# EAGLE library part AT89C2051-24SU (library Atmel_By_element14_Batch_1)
8-bit Microcontroller with 2K Bytes Flash
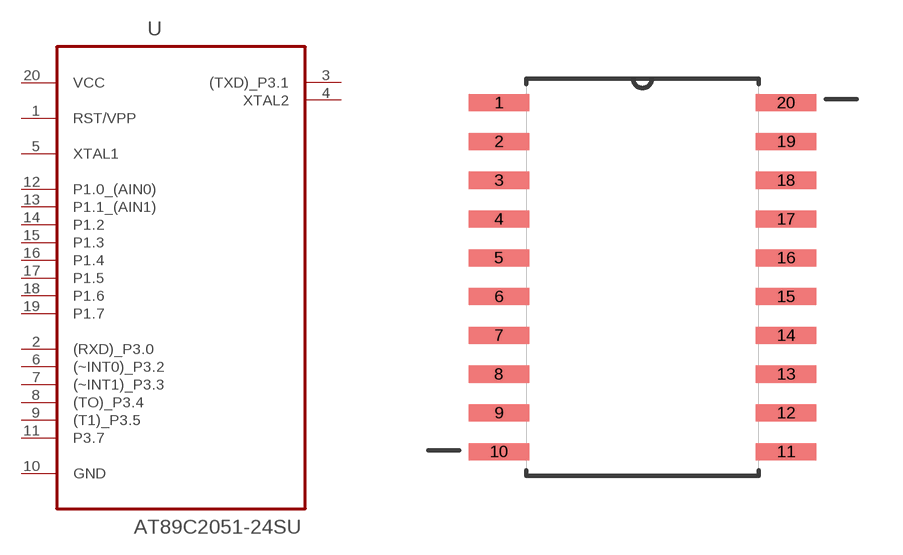
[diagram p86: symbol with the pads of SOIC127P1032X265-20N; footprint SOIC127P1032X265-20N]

Designator prefix U

## AT89C2051-24SU (DESCRIPTION: 8-bit Microcontroller with 2K Bytes Flash; MPN: AT89C2051-24SU; OC_FARNELL: 1715459; OC_NEWARK: 15R0321; PACKAGE: SOIC-20; SUPPLIER: Atmel)  [SOIC127P1032X265-20N]
1  RST/VPP  in
2  (RXD)_P3.0  in
3  (TXD)_P3.1  out
4  XTAL2  out
5  XTAL1  in
6  (~INT0)_P3.2  in
7  (~INT1)_P3.3  in
8  (TO)_P3.4  in
9  (T1)_P3.5  in
10  GND  pas
11  P3.7
12  P1.0_(AIN0)
13  P1.1_(AIN1)
14  P1.2
15  P1.3
16  P1.4
17  P1.5
18  P1.6
19  P1.7
20  VCC  pwr

## Footprint SOIC127P1032X265-20N (pad centres in mm)
smd 1.981 x 0.559: 1 -4.699,5.715; 2 -4.699,4.445; 3 -4.699,3.175; 4 -4.699,1.905; 5 -4.699,0.635; 6 -4.699,-0.635; 7 -4.699,-1.905; 8 -4.699,-3.175; 9 -4.699,-4.445; 10 -4.699,-5.715; 11 4.699,-5.715; 12 4.699,-4.445; 13 4.699,-3.175; 14 4.699,-1.905; 15 4.699,-0.635; 16 4.699,0.635; 17 4.699,1.905; 18 4.699,3.175; 19 4.699,4.445; 20 4.699,5.715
